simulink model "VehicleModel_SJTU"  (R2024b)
settings: Solver=ode4  StartTime=0.0  StopTime=150  FixedStep=0.0001  RelTol=1e-3
model workspace (MAT data in the model file):
  Brake_MC_D = 3.3
  CarSimTCKMAP = [0.006425 0.006425 0.006425 0.006425 0.006424 0.006419 0.006386 0.006243 0.005735 0.004185 0.002578 0.000614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]
  CarSimTCLambdaPMAP = [1.864 1.78 1.701 1.608 1.56 1.519 1.464 1.412 1.356 1.309 1.259 1.203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]
  CarSimTCiMAP1 = [0 0.1 0.2 0.3 0.4 0.5 0.6 0.7 0.8 0.9 0.95 0.99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]
  CarSimTCiMAP2 = [0 0.102 0.202 0.306 0.353 0.4 0.452 0.502 0.551 0.6 0.65 0.7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]
  DOWN_Data_lookup = [0 0 0 0 0 0 0 0 0 0 0 0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]
  DOWN_Gear_lookup = [1 2 3 4 5]
  DOWN_Throttle_lookup = [0 1 2 3 4 5 6 7 8 9 10 11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]
  Diff_gear_ratio = 4.1
  MC_lever_ratio = 0.02381
  UP_Data_lookup = [13.2140963951 13.2140963951 13.2140963951 13.2140963951 13.2140963951 13.2140963951 13.6741047457 14.0455395451 14.3574336302 14.6810803701 15.0507893957 16.3806466373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]
  UP_Gear_lookup = [1 2 3 4 5]
  UP_Throttle_lookup = [0 1 2 3 4 5 6 7 8 9 10 11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]
  eng_One_Order_T = 0.005
  eng_T = [0 0 0 0 0 0 0 0 0 0 15 64.064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]
  eng_Ted = 0.005
  eng_n = [0 86.6667 173.333 433.333 750 866.667 1300 1733.33 2166.67 2600 3033.33 3466.67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]
  eng_throttle = [0 0.1 0.15 0.2 0.35 0.5 0.7 0.85 0.95 1]
  rotational_inertia_of_crankshaft = 0.16
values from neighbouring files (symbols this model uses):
  acc = data(2)    [control_simulink.m]    (also in init.m = 2; tempScript.m = 0; test.m = 1)
  gear = data(1)    [control_simulink.m]    (also in init.m = 1; tempScript.m = 2)
  slope = data(5)    [control_simulink.m]    (also in init.m = -0.3; tempScript.m = -0.2)
  steer = data(3)    [control_simulink.m]    (also in init.m = 0; tempScript.m = 0; test.m = steer+0.01)
  v0 = 0    [init.m]    (also in tempScript.m = 3.505)
  x0 = -27.92254    [init.m]    (also in tempScript.m = 383.713846257)
  y0 = 292.5054    [init.m]    (also in tempScript.m = -781.380679998)
  yaw = -1.3    [init.m]    (also in tempScript.m = -1.125)
undefined symbols (not defined in the file or in its folder): VehicleModel_SJTU

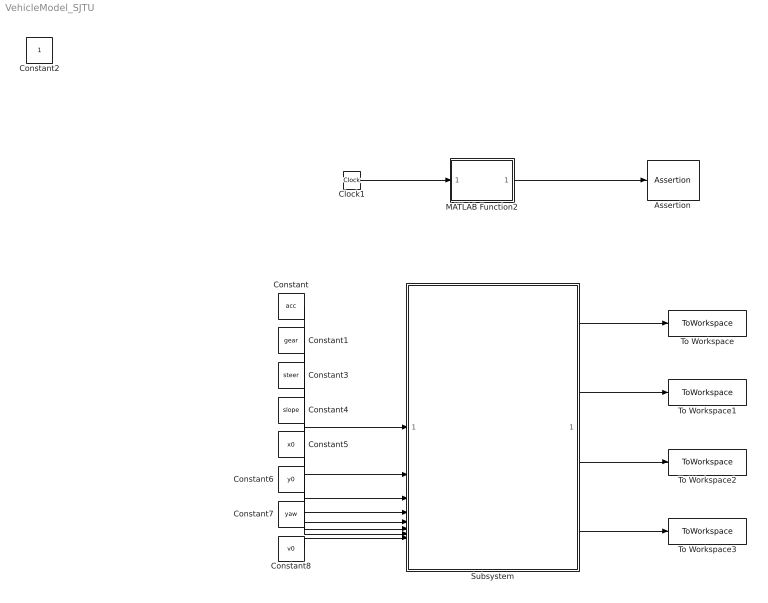
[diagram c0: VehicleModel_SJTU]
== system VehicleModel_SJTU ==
  Assertion : Assertion  AssertionFailFcn=set_param(VehicleModel_SJTU,'SimulationCommand', 'pause')  StopWhenAssertionFail=off
  Clock1 : Clock
  Constant : Constant  Value=acc
  Constant1 : Constant  Value=gear
  Constant3 : Constant  Value=steer
  Constant4 : Constant  Value=slope
  Constant5 : Constant  Value=x0
  Constant6 : Constant  Value=y0
  Constant7 : Constant  Value=yaw
  Constant8 : Constant  Value=v0
  MATLAB Function2 : MATLAB Function  TreatAsAtomicUnit=on
  Subsystem : ModelReference  ModelNameDialog=Subsystem0  ModelReferenceVersion=11.13  CopyOfModelProtected=on
  To Workspace : ToWorkspace  VariableName=phi  SaveFormat=Timeseries  SampleTime=-1
  To Workspace1 : ToWorkspace  VariableName=x  SaveFormat=Timeseries  SampleTime=-1
  To Workspace2 : ToWorkspace  VariableName=y  SaveFormat=Timeseries  SampleTime=-1
  To Workspace3 : ToWorkspace  VariableName=velocity  SaveFormat=Timeseries  SampleTime=-1
  Constant2 : Constant  IOType=siggen
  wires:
  Clock1/1 -> MATLAB Function2/1(u)
  MATLAB Function2/1(y) -> Assertion/1
  Subsystem/1 -> To Workspace/1
  Subsystem/2 -> To Workspace1/1
  Subsystem/3 -> To Workspace2/1
  Subsystem/4 -> To Workspace3/1
  Constant/1 -> Subsystem/1
  Constant1/1 -> Subsystem/2
  Constant3/1 -> Subsystem/3
  Constant4/1 -> Subsystem/4
  Constant5/1 -> Subsystem/5
  Constant6/1 -> Subsystem/6
  Constant7/1 -> Subsystem/7
  Constant8/1 -> Subsystem/8

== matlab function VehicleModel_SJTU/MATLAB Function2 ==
function y = fcn(u)
if u==0.1
    y=0;
else
    y = 1;
end
